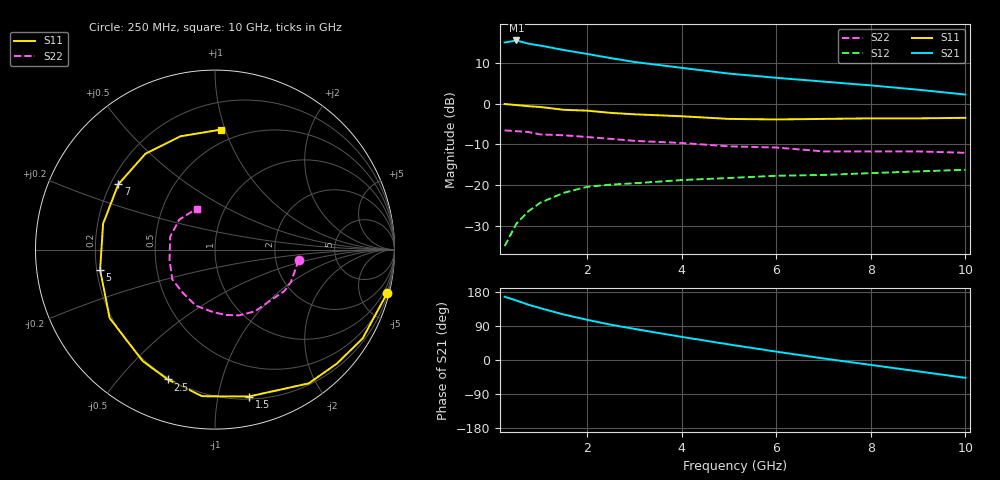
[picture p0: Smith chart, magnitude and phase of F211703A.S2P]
!ATF-21170
!S-PARAMETERS at Vds=3V  Id=20mA.  LAST UPDATED 07-22-92
# ghz s ma r 50
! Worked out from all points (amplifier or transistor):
!   15 points, 250 MHz to 10 GHz, reference 50 ohm
!   highest |S21| = 15.5 dB at 500 MHz (marker M1)
!   |S21| within 3 dB of that: start of sweep to 1.84 GHz
!   unconditionally stable (mu >= 1): 6.567 GHz to end of sweep
!   at 750 MHz: K = 0.23, MSG = 20.5 dB, |S12| = -26.4 dB
!   at 3 GHz: K = 0.56, MSG = 14.8 dB, |S12| = -19.5 dB
!   at 10 GHz: K = 1.31, MAG = 5.8 dB, |S12| = -16.2 dB
!   lowest NFmin = 0.40 dB at 500 MHz
!   S11 on the Smith chart (normalised r, x): 250 MHz: 0.34, -8.13; 1.5 GHz: 0.22, -1.23; 2.5 GHz: 0.19, -0.68; 5 GHz: 0.21, -0.08; 7 GHz: 0.23, +0.29; 10 GHz: 0.40, +0.97
0.25  0.99 -14.0  5.61 167.0  0.018 79.0  0.47 -7.0
0.5  0.96 -31.0  5.93 157.0  0.034 72.0  0.46 -23.0
0.75  0.93 -43.0  5.42 146.0  0.048 65.0  0.45 -31.0
1  0.91 -55.0  5.14 137.0  0.061 56.0  0.42 -42.0
1.5  0.84 -77.0  4.53 120.0  0.081 44.0  0.41 -57.0
2  0.82 -95.0  4.05 106.0  0.096 36.0  0.39 -70.0
2.5  0.77 -110.0  3.6 93.0  0.102 27.0  0.37 -80.0
3  0.74 -123.0  3.23 82.0  0.106 21.0  0.35 -91.0
4  0.7 -147.0  2.74 61.0  0.116 9.0  0.33 -109.0
5  0.65 -170.0  2.33 41.0  0.123 -1.0  0.3 -127.0
6  0.64 167.0  2.07 22.0  0.131 -10.0  0.29 -145.0
7  0.65 146.0  1.86 4.0  0.134 -17.0  0.26 -167.0
8  0.66 126.0  1.67 -13.0  0.141 -28.0  0.26 164.0
9  0.66 107.0  1.48 -30.0  0.148 -39.0  0.26 140.0
10  0.67 87.0  1.29 -47.0  0.155 -50.0  0.25 114.0
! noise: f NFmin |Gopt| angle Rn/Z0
0.5  0.4  0.93  17  0.9
1  0.5  0.85  35  0.7
2  0.6  0.7  70  0.46
4  0.9  0.59  148  0.14
6  1.2  0.54  -177  0.09
